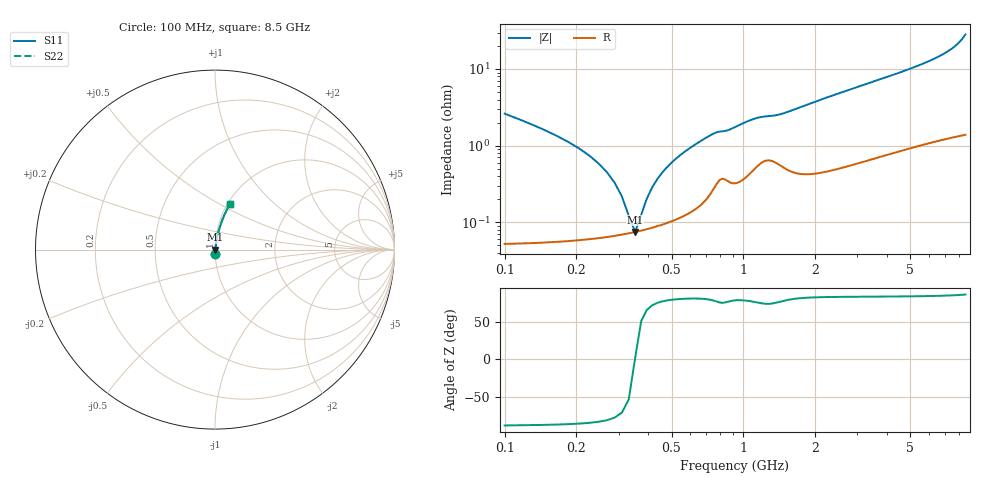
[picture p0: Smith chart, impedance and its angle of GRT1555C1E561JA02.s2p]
!Murata Part Number: GRT1555C1E561JA02
!These Parameters are Measured in Series Mode Connection
!Data Generated on Jun 19, 2026
!  o--ll--o
!Port1  Port2
!  o------o
!Operation Temp=25[degC], DC Bias Voltage=0[V]
!Freq. Start=100[MHz] Stop=9[GHz] 401[Steps]
# Hz S RI R 50
!Freq.(Hz) S11(Real) S11(Imag) S21(Real) S21(Imag) S12(Real) S12(Imag) S22(Real) S22(Imag)
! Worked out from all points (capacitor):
!   401 points, 100 MHz to 8.5 GHz, reference 50 ohm
!   read as one part in series: C = 559 pF near 142 MHz
!   lowest |Z| = 74.3 mohm at 352 MHz (marker M1)
!   series resonance near 351.5 MHz, so ESL is about 370 pH
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1e8  0.0012 -0.0261  0.9988 0.0261  0.9988 0.0261  0.0012 -0.0261
1.42e8  0.000819 -0.0167  0.9992 0.0167  0.9992 0.0167  0.000819 -0.0167
2.26e8  0.000652 -0.00738  0.9993 0.00738  0.9993 0.00738  0.000652 -0.00738
2.68e8  0.000658 -0.00445  0.9993 0.00445  0.9993 0.00445  0.000658 -0.00445
3.1e8  0.00069 -0.00204  0.9993 0.00204  0.9993 0.00204  0.00069 -0.00204
3.31e8  0.000714 -0.000977  0.9993 0.000977  0.9993 0.000977  0.000714 -0.000977
3.52e8  0.000743 2.23e-05  0.9993 -2.23e-05  0.9993 -2.23e-05  0.000743 2.23e-05
3.73e8  0.000775 0.000965  0.9992 -0.000965  0.9992 -0.000965  0.000775 0.000965
3.94e8  0.000811 0.00186  0.9992 -0.00186  0.9992 -0.00186  0.000811 0.00186
4.36e8  0.000896 0.00354  0.9991 -0.00354  0.9991 -0.00354  0.000896 0.00354
4.99e8  0.00106 0.00585  0.9989 -0.00585  0.9989 -0.00585  0.00106 0.00585
5.83e8  0.00135 0.00872  0.9987 -0.00872  0.9987 -0.00872  0.00135 0.00872
7.09e8  0.00225 0.0128  0.9978 -0.0128  0.9978 -0.0128  0.00225 0.0128
1.108e9  0.00532 0.0216  0.9947 -0.0216  0.9947 -0.0216  0.00532 0.0216
1.507e9  0.0056 0.0263  0.9944 -0.0263  0.9944 -0.0263  0.0056 0.0263
2.116e9  0.00596 0.0394  0.994 -0.0394  0.994 -0.0394  0.00596 0.0394
2.914e9  0.00873 0.0553  0.9913 -0.0553  0.9913 -0.0553  0.00873 0.0553
4.3e9  0.015 0.083  0.985 -0.083  0.985 -0.083  0.015 0.083
5.707e9  0.0237 0.1147  0.9763 -0.1147  0.9763 -0.1147  0.0237 0.1147
7.114e9  0.0383 0.1588  0.9617 -0.1588  0.9617 -0.1588  0.0383 0.1588
7.891e9  0.055 0.1991  0.945 -0.1991  0.945 -0.1991  0.055 0.1991
8.5e9  0.0848 0.2551  0.9152 -0.2551  0.9152 -0.2551  0.0848 0.2551
